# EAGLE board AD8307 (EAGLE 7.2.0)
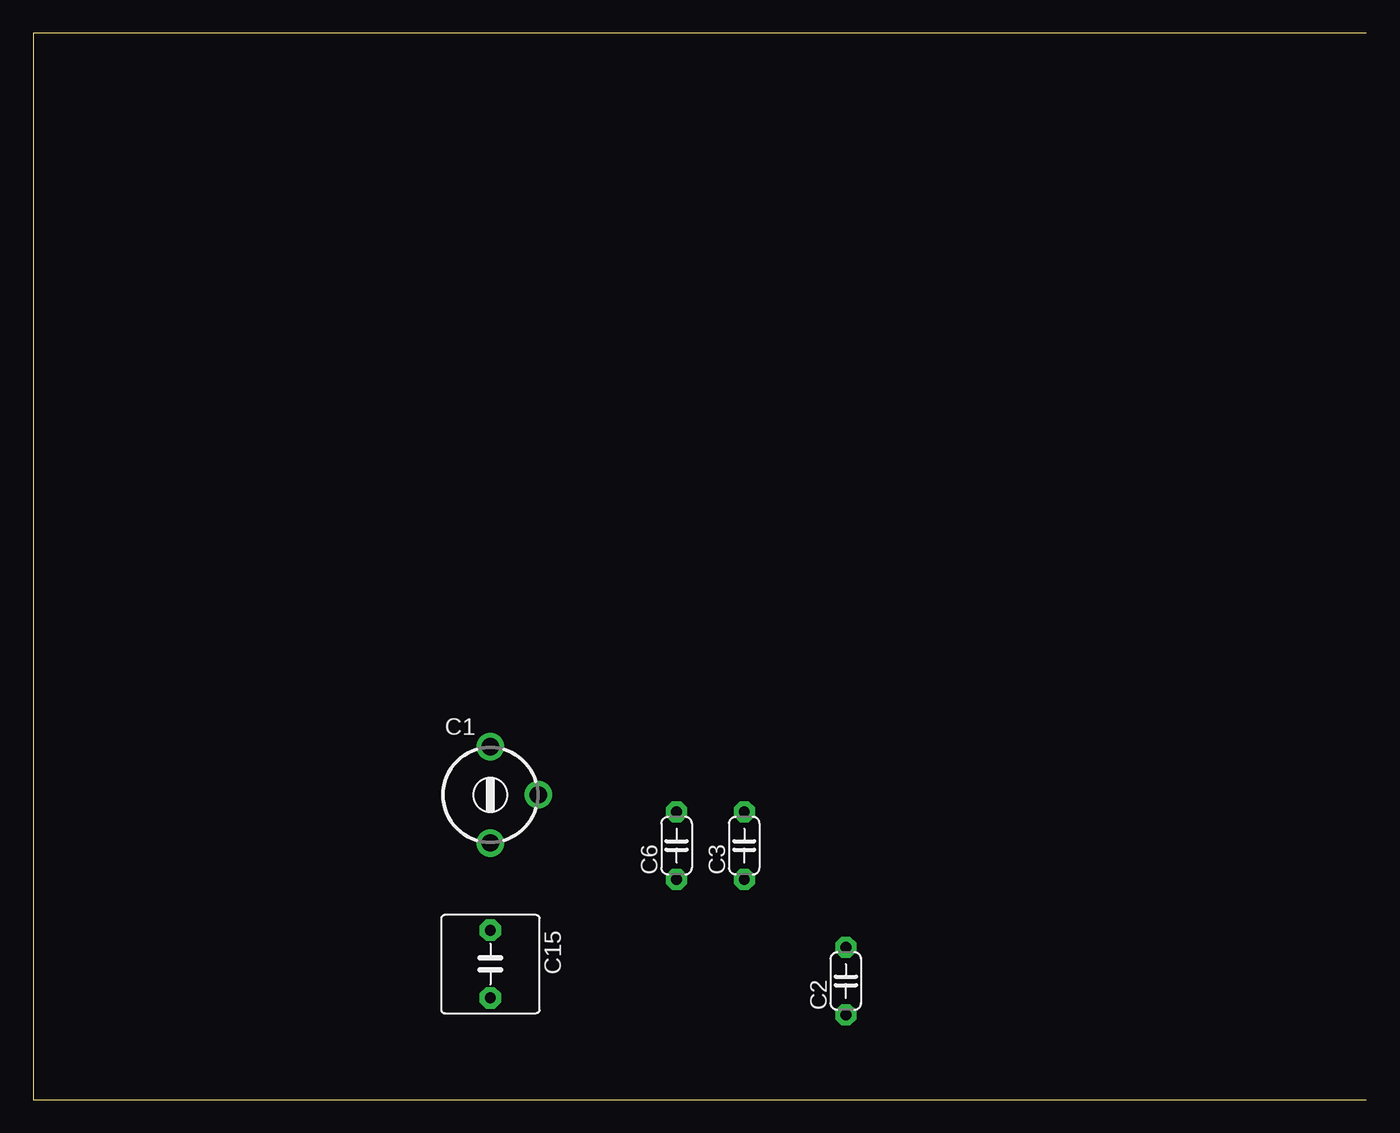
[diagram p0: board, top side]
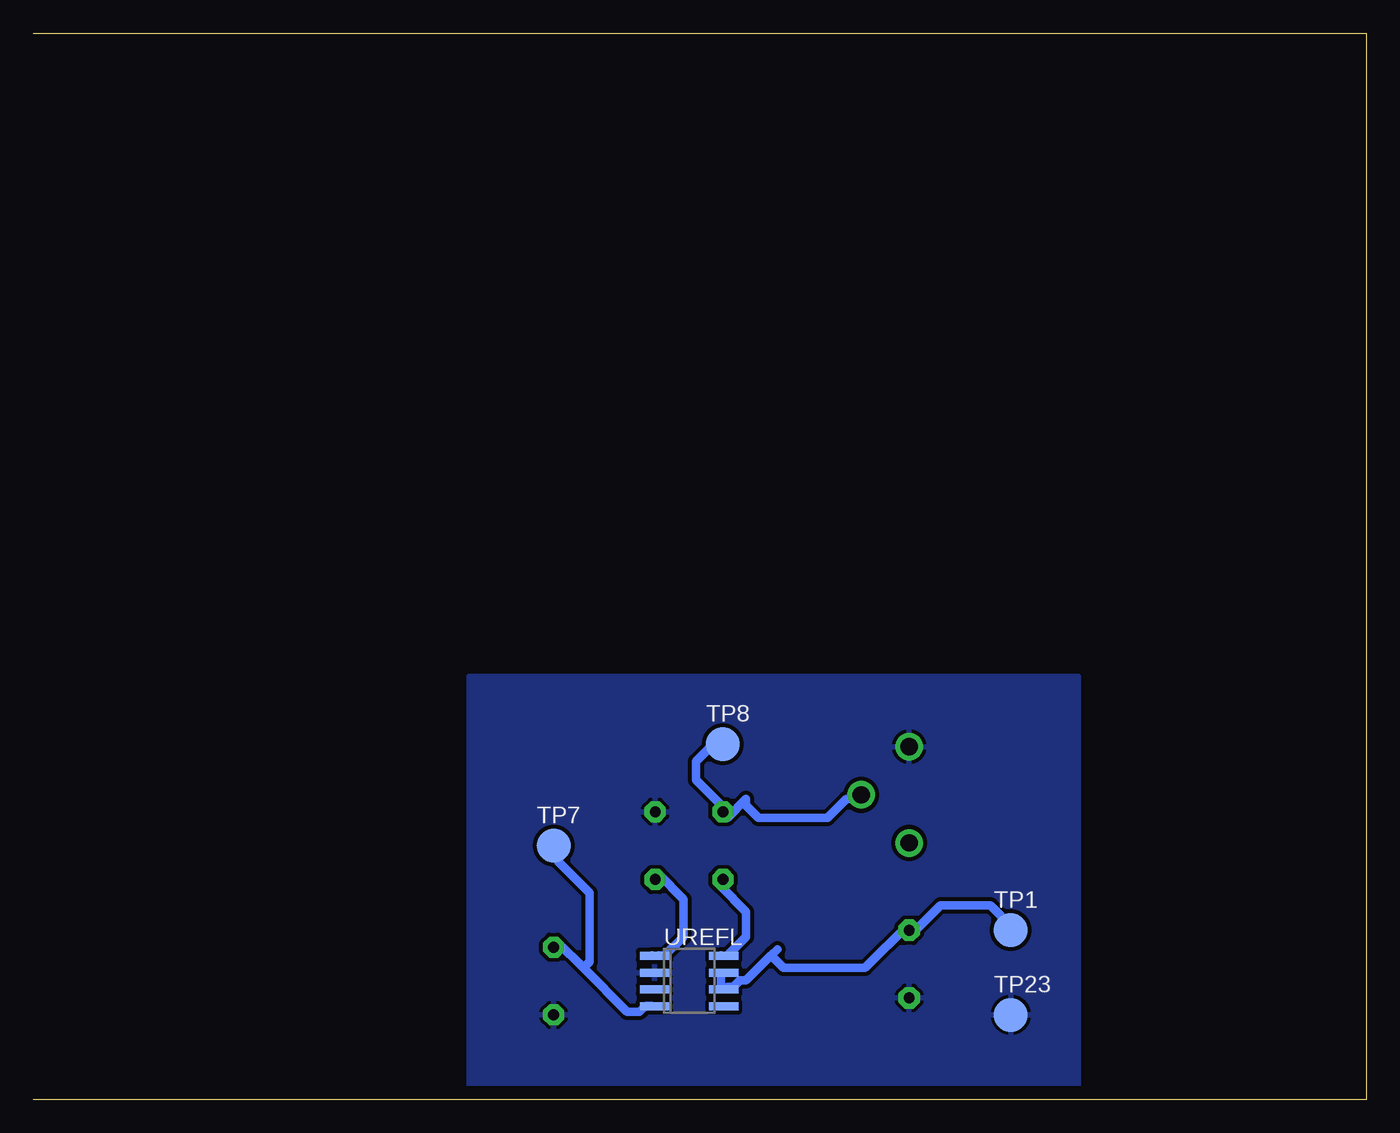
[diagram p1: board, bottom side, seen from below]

Size 100 x 80 mm. Coordinates in mm from the lower left corner, seen from the top.
Outline: 100,0 0,0 0,80 100,80
Copper layers (1*16): Top 0.035mm / dielectric 1.5mm / Bottom 0.035mm
Design rules "Power Meter *": minimum track width 25mil, minimum drill 50mil, track to track 12mil, track to pad 12mil, pad to pad 12mil, via to via 0.205mm, smd to smd 10mil, copper to edge 40mil, drill to drill 8mil, minimum pad ring 15mil, minimum via ring 12mil, stop-mask expansion 0.4mm, vias tented up to drill 0mil, thermal gap 10mil

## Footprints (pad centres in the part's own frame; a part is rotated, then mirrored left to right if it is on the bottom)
CTRIM808-BC = drill 1.3: 1 -3.607,0; 2 0,3.607; 3 3.607,0
C050-024X044 = drill 0.813 octagon: 1 -2.54,0; 2 2.54,0
C5B7.2 = drill 0.813 pad 1.6 octagon: 1 -2.54,0; 2 2.54,0
B2,54 = smd 2.54 x 2.54: TP 0,0
SO08 = smd 0.6 x 2.2: 1 -1.905,-2.6; 2 -0.635,-2.6; 3 0.635,-2.6; 4 1.905,-2.6; 5 1.905,2.6; 6 0.635,2.6; 7 -0.635,2.6; 8 -1.905,2.6

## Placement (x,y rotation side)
C1  22p  [CTRIM808-BC]  34.29,22.86 270 top
C2  10n  [C050-024X044]  60.96,8.89 90 top
C3  100n  [C050-024X044]  53.34,19.05 90 top
C6  100n  [C050-024X044]  48.26,19.05 90 top
C15  10ÃÂµ  [C5B7.2]  34.29,10.16 270 top
TP1  PTR1B2,54  [B2,54]  26.67,12.7 0 bottom
TP7  PTR1B2,54  [B2,54]  60.96,19.05 0 bottom
TP8  PTR1B2,54  [B2,54]  48.26,26.67 0 bottom
TP23  PTR1B2,54  [B2,54]  26.67,6.35 0 bottom
UREFL  AD8307SO8  [SO08]  50.8,8.89 270 bottom

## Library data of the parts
C1-C3 C6 = resistor
C15 = capacitor-wima
TP1 TP7 TP8 TP23 = testpad
UREFL = -- Eigene

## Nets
GND: C1.1 C2.1 C3.2 C15.2 TP23.TP UREFL.2
N$14: C3.1 UREFL.1
N$15: C1.2 C6.2 TP8.TP
N$16: C6.1 UREFL.8
N$28: C2.2 TP7.TP UREFL.4
N$42: C15.1 TP1.TP UREFL.6 UREFL.7

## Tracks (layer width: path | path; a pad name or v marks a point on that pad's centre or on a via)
GND
  pour Bottom: 21.59,31.75 67.31,31.75 67.31,0 21.59,0
N$14
  Bottom 0.635: 53.57,10.81 UREFL.1 53.1,10.81 52.63,10.81 51.22,12.22 51.22,15.04 53.1,16.92 C3.1 53.57,16.45
N$15
  Bottom 0.635: C1.2 38.06,22.55 39,22.55 40.41,21.14 45.58,21.14 46.52,22.09 46.52,22.55 47.93,21.14 C6.2 47.93,21.61 50.28,23.96 50.28,25.38 49.34,26.31 48.4,26.31 TP8.TP
N$16
  Bottom 0.635: 48.4,10.81 UREFL.8 47.93,10.81 46.52,12.22 46.52,14.1 48.4,15.98 48.4,16.45 C6.1
N$28
  Bottom 0.635: 58.74,9.87 60.62,11.75 C2.2 | 58.74,9.87 55.45,6.58 54.51,6.58 54.04,7.05 53.57,7.05 UREFL.4 | 58.74,9.87 58.27,10.34 58.27,15.51 60.62,17.86 60.62,18.8 TP7.TP
N$42
  Bottom 0.635: UREFL.7 48.4,9.4 48.4,8.46 UREFL.6 47.93,8.46 47.46,8.46 46.99,8.93 46.52,8.93 44.64,10.81 | 44.17,11.28 44.64,10.81 | TP1.TP 26.78,13.16 28.19,14.57 31.95,14.57 33.83,12.69 C15.1 34.3,13.16 37.59,9.87 43.7,9.87 44.64,10.81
